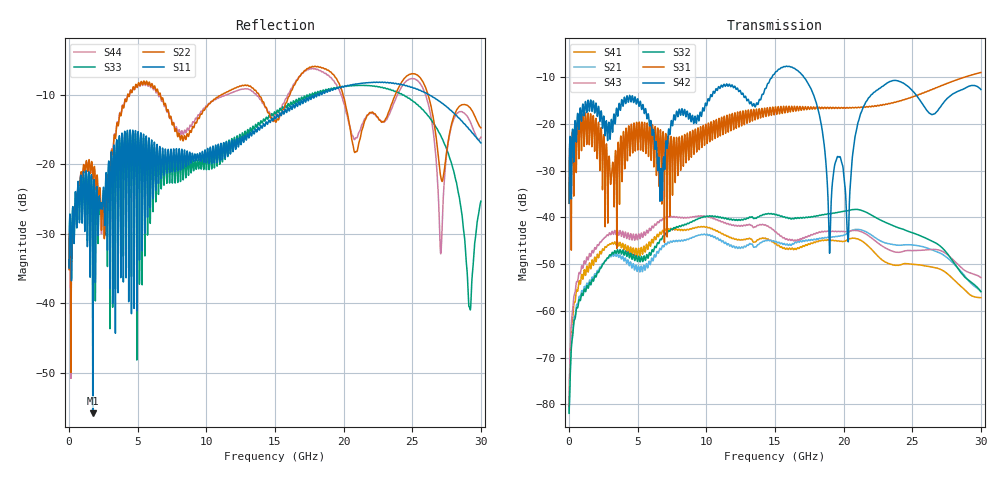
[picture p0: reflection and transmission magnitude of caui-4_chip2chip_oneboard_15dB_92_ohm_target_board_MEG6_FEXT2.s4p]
! Touchstone file from project caui-4_chip2chip_oneboard
! Exported from Circuit Design 8.0.0
! Variables:
!  $ModelNames_Index = 0
!  $ModelNames_Index1 = 0
!  $ModelNames_Index2 = 0
!  $ModelNames_Index3 = 0
!  $ModelNames_Index4 = 0
!  $ModelNames_Index5 = 0
!  Lbo = 0.5in
!  Lmain = 16in
!  lcap = 0.25in
# GHZ S MA R 50.000000
! Modal data exported
! Port[1] = Port1
! Port[2] = Port2
! Port[3] = Port3
! Port[4] = Port4
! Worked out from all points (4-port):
!   3000 points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, 10 MHz to 30 GHz, reference 50 ohm
!   strongest paths, dB at 10 MHz, 7.51 GHz, 15.01 GHz, 22.51 GHz, 30 GHz:
!     S42: -36.9, -20.0, -9.0, -12.6, -12.6
!     S31: -37.0, -29.1, -16.6, -16.0, -9.0
!     S32: -81.9, -42.6, -39.4, -40.3, -55.9
!     S43: -80.5, -39.9, -43.0, -45.5, -52.9
!     S21: -81.7, -45.3, -45.3, -44.7, -55.8
!     S41: -81.1, -42.7, -45.6, -48.3, -57.2
!   lowest |S11| = -55.8 dB at 1.73 GHz (marker M1), VSWR 1.00, Z = 50.1 + j0.149 ohm
!   |S11| at or under -10 dB: start of sweep to 17.9 GHz; 17.95 GHz to 18.07 GHz (121.1 MHz wide, 0.672 % of centre); 26.25 GHz to end of sweep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
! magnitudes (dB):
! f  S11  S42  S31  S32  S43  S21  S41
! 10 MHz  -34.9  -36.9  -37.0  -81.9  -80.5  -81.7  -81.1
! 1.73 GHz  -55.8  -15.9  -19.6  -53.4  -47.3  -52.9  -49.6
! 6.71 GHz  -22.0  -29.5  -24.4  -44.8  -40.7  -46.9  -43.6
! 16.33 GHz  -11.4  -8.0  -17.3  -40.3  -45.0  -45.7  -46.8
! 20.3 GHz  -8.6  -43.9  -16.5  -38.6  -43.0  -43.3  -44.8
! 22.09 GHz  -8.2  -13.6  -16.1  -39.6  -44.5  -43.9  -47.0
! 30 GHz  -16.9  -12.6  -9.0  -55.9  -52.9  -55.8  -57.2
